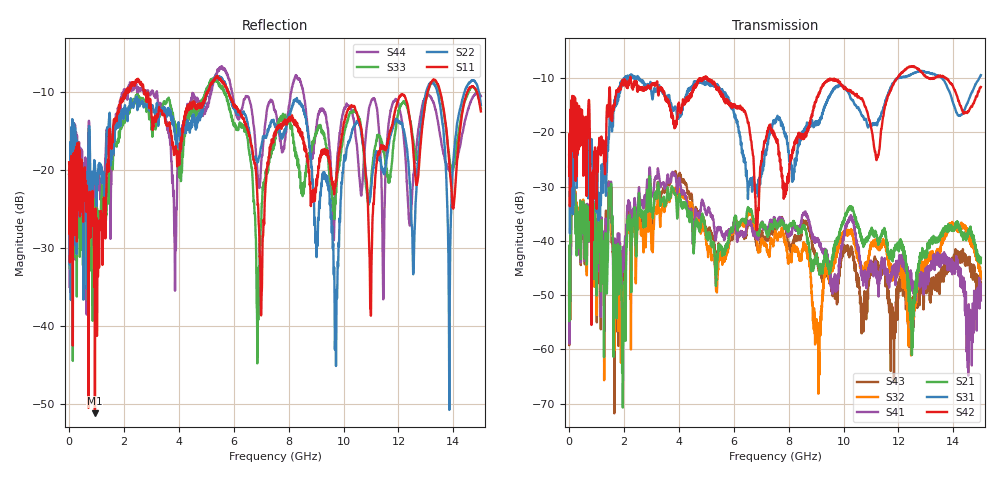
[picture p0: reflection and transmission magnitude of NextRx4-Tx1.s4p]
! FILE: N:\QM 2007\Prüfprotokolle\Highspeed\Konfektionierte Ltg\L45593-D106\D30\8216\0002\Next  Platine 1\NextRx4-Tx1.s4p
# MHz S DB R 50.00
! FREQ  S11  S12  S13  S14
!  S21  S22  S23  S24
!  S31  S32  S33  S34
!  S41  S42  S43  S44
!  DB  ANG  DB  ANG  DB  ANG  DB  ANG
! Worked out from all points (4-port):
!   2999 points, 10 MHz to 15 GHz, reference 50 ohm
!   strongest paths, dB at 10 MHz, 3.755 GHz, 7.505 GHz, 11.26 GHz, 15 GHz:
!     S42: -26.3, -16.5, -20.7, -24.2, -11.6
!     S31: -24.2, -15.3, -18.3, -18.0, -9.4
!     S21: -47.4, -29.9, -36.6, -39.8, -43.1
!     S41: -49.2, -27.5, -36.0, -46.7, -51.0
!     S32: -47.8, -30.2, -38.3, -41.6, -47.0
!     S43: -49.6, -27.6, -36.5, -43.9, -47.9
!   lowest |S11| = -51.1 dB at 950 MHz (marker M1), VSWR 1.01, Z = 49.8 - j0.2 ohm
!   |S11| at or under -10 dB: start of sweep to 2.07 GHz; 2.782 GHz to 5.045 GHz (2.262 GHz wide, 57.8 % of centre); 5.816 GHz to 13.06 GHz (7.242 GHz wide, 76.7 % of centre)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
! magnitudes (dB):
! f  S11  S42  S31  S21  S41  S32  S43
! 10 MHz  -19.0  -26.3  -24.2  -47.4  -49.2  -47.8  -49.6
! 950 MHz  -51.1  -23.1  -25.2  -32.9  -33.3  -34.3  -35.0
! 8.315 GHz  -14.1  -21.4  -24.0  -38.0  -37.5  -41.8  -39.4
! 9.71 GHz  -21.4  -10.4  -11.7  -40.3  -48.7  -42.6  -49.4
! 10.43 GHz  -12.2  -13.2  -14.9  -36.0  -38.8  -41.0  -45.4
! 13.85 GHz  -19.2  -10.7  -12.5  -37.8  -43.3  -36.7  -43.3
! 15 GHz  -12.5  -11.6  -9.4  -43.1  -51.0  -47.0  -47.9
